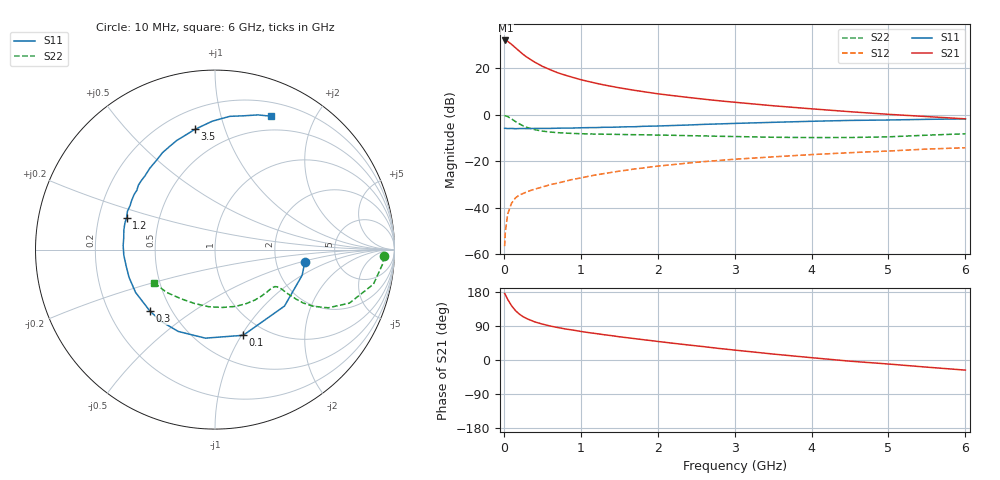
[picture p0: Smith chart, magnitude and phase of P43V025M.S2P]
! SIEMENS Small Signal Semiconductors
! BFP182
! Si NPN RF Bipolar Junction Transistor in SOT143
! VCE = 3 V  IC = 25 mA
! Common Emitter S-Parameters:  March  1996
# GHz  S  MA  R  50
!  f  S11  S21  S12  S22
! GHz  MAG  ANG  MAG  ANG  MAG  ANG  MAG  ANG
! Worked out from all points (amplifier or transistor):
!   36 points, 10 MHz to 6 GHz, reference 50 ohm
!   highest |S21| = 31.8 dB at 20 MHz (marker M1)
!   |S21| within 3 dB of that: start of sweep to 146.4 MHz
!   unconditionally stable (mu >= 1): 581.3 MHz to 5.469 GHz
!   at 250 MHz: K = 0.61, MSG = 29.8 dB, |S12| = -33.9 dB
!   at 1.4 GHz: K = 1.25, MAG = 15.4 dB, |S12| = -24.8 dB
!   at 6 GHz: K = 0.95, MSG = 6.2 dB, |S12| = -14.3 dB
!   S11 on the Smith chart (normalised r, x): 10 MHz: 2.93, -0.54; 100 MHz: 0.80, -1.02; 300 MHz: 0.38, -0.34; 1.2 GHz: 0.32, +0.16; 3.5 GHz: 0.32, +0.80; 6 GHz: 0.34, +1.45
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0.01  0.5053 -7.8  38.73 175.7  0.0015 83.5  0.9417 -2.2
0.02  0.5062 -16.4  38.75 172.0  0.0031 80.4  0.9376 -4.9
0.05  0.4989 -39.1  37.08 159.9  0.0073 77.4  0.9036 -12.3
0.1  0.5026 -71.8  31.98 143.3  0.0125 62.4  0.8064 -21.7
0.15  0.4963 -96.2  27.11 130.6  0.0162 56.4  0.7094 -27.2
0.2  0.4998 -114.2  22.96 121.3  0.0187 54.0  0.6313 -30.0
0.25  0.5002 -127.0  19.51 114.3  0.0202 50.8  0.5729 -31.2
0.3  0.4984 -136.9  16.96 109.1  0.022 51.3  0.5287 -31.4
0.4  0.5028 -151.7  13.32 100.7  0.0251 50.8  0.4738 -31.2
0.5  0.5033 -162.2  10.83 94.8  0.0278 51.7  0.4406 -30.8
0.6  0.5034 -169.7  9.171 89.8  0.0312 52.9  0.4213 -30.6
0.7  0.509 -176.5  7.859 85.7  0.0338 54.7  0.4081 -30.8
0.8  0.5122 177.4  6.96 81.9  0.0371 55.1  0.3992 -31.2
1.1  0.5232 163.8  5.107 72.4  0.0473 56.1  0.3833 -33.8
1.2  0.5239 160.1  4.677 69.7  0.0507 56.1  0.3804 -35.0
1.7  0.5466 142.8  3.3 56.4  0.068 54.6  0.3689 -42.4
2.2  0.5812 128.6  2.538 44.2  0.0843 51.5  0.3584 -51.6
2.8  0.6285 113.6  1.968 30.4  0.1037 46.4  0.341 -64.6
3.5  0.6796 99.4  1.54 15.7  0.1235 40.1  0.3251 -82.5
4.5  0.7469 83.7  1.148 -3.1  0.1517 31.5  0.3211 -110.9
5.5  0.7878 72.3  0.903 -18.9  0.1815 23.0  0.3602 -138.6
6  0.8056 67.3  0.807 -26.7  0.1938 17.9  0.386 -151.3
